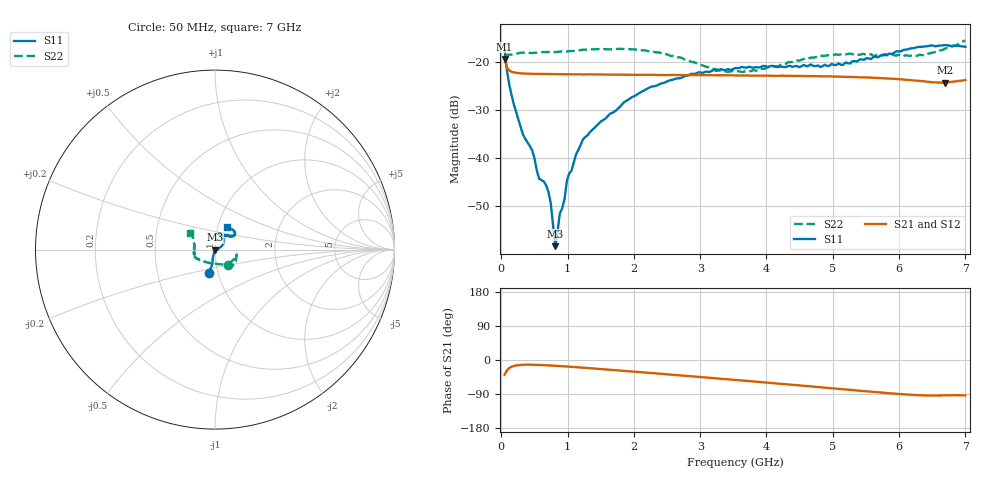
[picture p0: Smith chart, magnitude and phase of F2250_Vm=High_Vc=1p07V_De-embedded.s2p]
! Integrated Device Technology
! Corporate Headquarters
! 6024 Silver Creek Valley Road
! San Jose, CA 95138  USA
! Phone:  1-408-284-8200
! Toll Free:  1-800-223-1366
! Webpage:  http://www.idt.com/
! Timing and RF Division
! 515 Groton Road, Suite 102
! Westford, MA 01886-6024
! Device:  F2250
! Description: Voltage Variable RF Attenuator
! Frequency:  50.0 -  6000.00 MHz
! Package:  3x3 mm Thin QFN Plastic Package: 16 pin
! Ports:  2 RF, 3 DC
!  Pin  1  = GND
!  Pin  2  = NC
!  Pin  3  = RF1  = Port 1
!  Pin  4  = NC
!  Pin  5  = GND
!  Pin  6  = GND
!  Pin  7  = GND
!  Pin  8  = GND
!  Pin  9  = NC
!  Pin 10  = RF2  = Port 2
!  Pin 11  = NC
!  Pin 12  = GND
!  Pin 13  = GND
!  Pin 14  = VCNTRL
!  Pin 15  = VDD
!  Pin 16  = VMODE
! Vcntrl:  1.070 Volts
! Vmode:  +3.300 Volts
! Vdd:  +3.30  Volts
! Current:  1.328 mA
! Data:  The device was measured on a the F2250 evaluation board which has
!  individual transmission lines to the RF pins.  Data was collected
!  using a calibrated network analyzer.  The evaluation board was
!  de-embedded using a TRL calibration technique.
!  The reference plane is the edge of the package pin.
! Misc:  SN 10
!  Action Tracker AT0258
! Date Measured:  2014-11-26
! Date:  2015-10-15  MJV
! Note:
!  Integrated Device Technology supplies this data as a sample of measured
!  data at the package pin for this product.  Your particular data for this
!  product may vary.
!  Data was taken at 25 degrees C.
!  Integrated Device Technology reserves the right to change this data at anytime.
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# GHz S dB R 50
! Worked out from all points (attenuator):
!   201 points, 50 MHz to 7 GHz, reference 50 ohm
!   highest |S21| = -19.41 dB at 50 MHz (marker M1); lowest = -24.3 dB at 6.687 GHz (marker M2)
!   lowest |S11| = -58.2 dB at 814.5 MHz (marker M3), VSWR 1.00, Z = 50.1 - j0.108 ohm
!   |S11| at or under -10 dB: start of sweep to end of sweep
!   |S22| runs from -22.1 to -15.5 dB; largest |S21 - S12| = 0.00032
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0.05  -17.39 -104.0  -19.41 -38.9  -19.41 -38.9  -18.96 -48.3
0.1195  -24.64 -102.8  -21.76 -21.4  -21.76 -21.4  -18.49 -18.2
0.29325  -33.63 -104.1  -22.37 -13.0  -22.38 -13.0  -18.08 -13.7
0.467  -38.37 -112.9  -22.46 -12.5  -22.47 -12.5  -18.15 -14.4
0.57125  -44.22 -109.5  -22.50 -13.0  -22.51 -13.1  -18.07 -16.7
0.64075  -44.79 -104.7  -22.50 -13.6  -22.51 -13.6  -17.95 -17.7
0.71025  -46.94 -96.2  -22.53 -14.2  -22.53 -14.2  -17.93 -19.4
0.745  -49.21 -88.9  -22.53 -14.6  -22.54 -14.6  -17.93 -20.0
0.8145  -58.24 -62.2  -22.56 -15.3  -22.56 -15.3  -17.96 -21.8
0.884  -51.38 -24.4  -22.54 -16.1  -22.53 -16.1  -17.86 -23.9
0.9535  -48.56 -34.9  -22.56 -16.8  -22.56 -16.8  -17.90 -24.9
0.98825  -44.76 -22.8  -22.56 -17.2  -22.56 -17.2  -17.85 -25.6
1.2315  -36.10 7.4  -22.60 -20.2  -22.58 -20.2  -17.45 -29.9
1.857  -28.31 25.7  -22.63 -28.7  -22.64 -28.7  -17.30 -38.0
2.37825  -24.66 37.5  -22.70 -36.0  -22.70 -36.0  -18.01 -44.9
2.86475  -22.47 50.6  -22.74 -43.0  -22.75 -43.0  -19.98 -56.8
3.525  -21.29 67.4  -22.79 -52.6  -22.81 -52.6  -22.02 -96.0
4.7065  -20.84 69.9  -22.94 -70.3  -22.95 -70.3  -19.10 -152.1
5.85325  -18.27 38.3  -23.45 -87.7  -23.44 -87.9  -18.66 -174.6
6.3745  -16.80 39.4  -24.02 -93.6  -24.03 -93.6  -18.64 166.5
6.68725  -16.52 46.6  -24.29 -93.2  -24.26 -93.4  -17.28 152.0
7  -16.85 61.9  -23.75 -93.4  -23.76 -93.5  -15.54 147.1
